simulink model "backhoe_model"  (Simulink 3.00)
settings: Solver=ode4  StartTime=0.0  StopTime=tfinal  FixedStep=T  RelTol=1e-3
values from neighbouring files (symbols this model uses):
  a1 = R(1,1)    [Jacobian.m]    (also in sub_static_vars.m = a(1))
  a2 = R(2,2)    [Jacobian.m]    (also in sub_static_vars.m = a(2))
  a3 = R(3,3)    [Jacobian.m]    (also in sub_static_vars.m = a(3))
  a4 = R(4,1)    [Jacobian.m]    (also in sub_static_vars.m = a(4))
  Ac = pi*(Dc.^2)/4    [cylinders.m]
  Ar = Ac-pi*(Dr.^2)/4    [cylinders.m]
  Cd = 2    [startup.m]
  dt = tfinal/N    (= 0.02)    [demo_trench.m]
  G1 = '0'    [sub_static_vars.m]    (also in symbolic_manip.m = G)
  G2 = char(G{2})    [sub_static_vars.m]    (also in symbolic_manip.m = G)
  G3 = char(G{3})    [sub_static_vars.m]    (also in symbolic_manip.m = G)
  G4 = char(G{4})    [sub_static_vars.m]    (also in symbolic_manip.m = G)
  Lcyl = [12.5*2 25 25.5 21.5]'    [cylinders.m]
  M11 = char(M{1})    [sub_static_vars.m]
  M12 = char(M{2})    [sub_static_vars.m]
  M13 = char(M{3})    [sub_static_vars.m]
  M14 = char(M{4})    [sub_static_vars.m]
  M21 = char(M{5})    [sub_static_vars.m]
  M22 = char(M{6})    [sub_static_vars.m]
  M23 = char(M{7})    [sub_static_vars.m]
  M24 = char(M{8})    [sub_static_vars.m]
  M31 = char(M{9})    [sub_static_vars.m]
  M32 = char(M{10})    [sub_static_vars.m]
  M33 = char(M{11})    [sub_static_vars.m]
  M34 = char(M{12})    [sub_static_vars.m]
  M41 = char(M{13})    [sub_static_vars.m]
  M42 = char(M{14})    [sub_static_vars.m]
  M43 = char(M{15})    [sub_static_vars.m]
  M44 = char(M{16})    [sub_static_vars.m]
  prelief = 2250    [backhoesim.m]
  pT = 0    [backhoesim.m]
  q0 = cyl_to_joint(yc0,R)    [backhoesim.m]
  qmax = cyl_to_joint([yclim(2,1) yclim(2,1) yclim(1,2) yclim(1,3) yclim(1,4)],R)    [backhoesim.m]    (also in demo_trench.m = [1.5708    1.0907    6.1403    6.5025])
  qmin = cyl_to_joint([yclim(1,1) yclim(1,1) yclim(2,2) yclim(2,3) yclim(2,4)],R)    [backhoesim.m]    (also in demo_trench.m = [-1.5708   -0.8529    3.6469    4.1089])
  QP = 33.11    [backhoesim.m]
  R1A = R(1,5)    [cyl_to_joint.m]    (also in dimensions.m = sqrt(R0N^2+(R01-RAN)^2); joint_to_cyl.m; SFr2taur.m; Sjoint_to_cyl.m)
  R1B = R(2,4)    [cyl_to_joint.m]    (also in dimensions.m = 35.875; joint_to_cyl.m; SFr2taur.m; Sjoint_to_cyl.m)
  R2C = R(2,3)    [cyl_to_joint.m]    (also in dimensions.m = 36; joint_to_cyl.m; SFr2taur.m; Sjoint_to_cyl.m)
  R2D = R(3,1)    [cyl_to_joint.m]    (also in dimensions.m = 9.875; joint_to_cyl.m; SFr2taur.m; Sjoint_to_cyl.m)
  R3F = R(3,5)-R(3,7)    [cyl_to_joint.m]    (also in dimensions.m = 4.5; joint_to_cyl.m; SFr2taur.m = R(3,8); Sjoint_to_cyl.m)
  R3G = R(4,2)    [cyl_to_joint.m]    (also in dimensions.m = 5.5; joint_to_cyl.m; SFr2taur.m; Sjoint_to_cyl.m)
  REF = R(3,6)    [cyl_to_joint.m]    (also in dimensions.m = 30.77; joint_to_cyl.m; SFr2taur.m; Sjoint_to_cyl.m)
  RFH = R(4,4)    [cyl_to_joint.m]    (also in dimensions.m = 9.5; joint_to_cyl.m; SFr2taur.m; Sjoint_to_cyl.m)
  RGH = R(4,5)    [cyl_to_joint.m]    (also in dimensions.m = 9.5; joint_to_cyl.m; SFr2taur.m; Sjoint_to_cyl.m)
  T = 0.001    [startup.m]
  T01A = R(1,12)    [cyl_to_joint.m]    (also in dimensions.m = atan(R0N/(R01-RAN)); joint_to_cyl.m; Sjoint_to_cyl.m)
  T12C = R(2,13)    [cyl_to_joint.m]    (also in dimensions.m = acos((R12^2+R2C^2-R1C^2)/(2*R12*R2C)); joint_to_cyl.m; Sjoint_to_cyl.m)
  T23D = acos((R23^2+R3D^2-R2D^2)/(2*R23*R3D))    [cyl_to_joint.m]    (also in dimensions.m; joint_to_cyl.m = R(3,14); SFr2taur.m = R(3,14); Sjoint_to_cyl.m = R(3,14))
  TB12 = R(2,12)    [cyl_to_joint.m]    (also in dimensions.m = acos((R1B^2+R12^2-R2B^2)/(2*R1B*R12)); joint_to_cyl.m; SFr2taur.m; Sjoint_to_cyl.m)
  TD23 = R(3,12)    [cyl_to_joint.m]    (also in dimensions.m = acos((R2D^2+R23^2-R3D^2)/(2*R2D*R23)); joint_to_cyl.m; SFr2taur.m; Sjoint_to_cyl.m)
  TDFE = R(3,13)    [cyl_to_joint.m]    (also in dimensions.m = acos((RDF^2+REF^2-RDE^2)/(2*RDF*REF)); joint_to_cyl.m; SFr2taur.m; Sjoint_to_cyl.m)
  TG34 = R(4,12)    [cyl_to_joint.m]    (also in dimensions.m = acos((R3G^2+R34^2-R4G^2)/(2*R3G*R34)); joint_to_cyl.m; SFr2taur.m; Sjoint_to_cyl.m)
  V1 = char(V{1})    [sub_static_vars.m]    (also in symbolic_manip.m = V)
  V2 = char(V{2})    [sub_static_vars.m]    (also in symbolic_manip.m = V)
  V3 = char(V{3})    [sub_static_vars.m]    (also in symbolic_manip.m = V)
  V4 = char(V{4})    [sub_static_vars.m]    (also in symbolic_manip.m = V)
  yc0 = [21.587 21.587 28.9 45.27 36.195]'    [backhoesim.m]
undefined symbols (not defined in the file or in its folder): Cc, Cr, den, K1, kd, Kr, num, pc0, pr0, td, wn, zeta
libraries: simulink3 x2
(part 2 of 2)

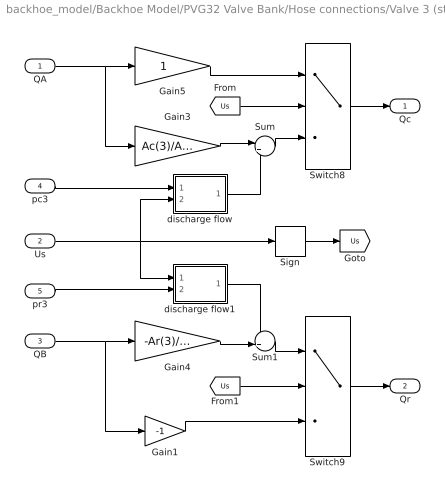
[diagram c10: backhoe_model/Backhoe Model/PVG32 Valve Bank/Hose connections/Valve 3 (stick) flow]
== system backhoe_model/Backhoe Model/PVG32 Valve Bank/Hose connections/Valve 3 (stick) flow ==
  QA : Inport  Port=1  PortWidth=-1  SampleTime=-1  DataType=auto
  Us : Inport  Port=2  PortWidth=-1  SampleTime=-1  DataType=auto
  QB : Inport  Port=3  PortWidth=-1  SampleTime=-1  DataType=auto
  pc3 : Inport  Port=4  PortWidth=-1  SampleTime=-1  DataType=auto
  pr3 : Inport  Port=5  PortWidth=-1  SampleTime=-1  DataType=auto
  Gain1 : Gain  Gain=-1  SaturateOnIntegerOverflow=on
  Gain3 : Gain  Gain=Ac(3)/Ar(3)  SaturateOnIntegerOverflow=on
  Gain4 : Gain  Gain=-Ar(3)/Ac(3)  SaturateOnIntegerOverflow=on
  Gain5 : Gain  Gain=1  SaturateOnIntegerOverflow=on
  Sign : Signum
  Sum : Sum  Inputs=|+-  SaturateOnIntegerOverflow=on
  Sum1 : Sum  Inputs=-+|  SaturateOnIntegerOverflow=on
  Switch8 : Switch  Threshold=0
  Switch9 : Switch  Threshold=0
  discharge flow : Subsystem
  discharge flow1 : Subsystem
  Qc : Outport  Port=1
  Qr : Outport  Port=2
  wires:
  [Us] -> Switch8/2
  Gain5/1 -> Switch8/1
  QA/1 -> Gain3/1, Gain5/1
  Switch8/1 -> Qc/1
  Sum/1 -> Switch8/3
  Gain3/1 -> Sum/1
  [Us] -> Switch9/2
  Gain1/1 -> Switch9/3
  QB/1 -> Gain4/1, Gain1/1
  Switch9/1 -> Qr/1
  Sum1/1 -> Switch9/1
  Gain4/1 -> Sum1/2
  discharge flow/1(Qd) -> Sum/2
  pr3/1 -> discharge flow1/2(p)
  pc3/1 -> discharge flow/1(p)
  Us/1 -> discharge flow/2(Us), discharge flow1/1(Us), Sign/1
  discharge flow1/1(Qd) -> Sum1/1
  Sign/1 -> [Us]

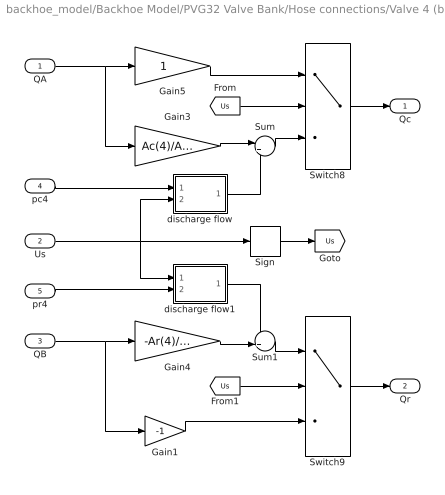
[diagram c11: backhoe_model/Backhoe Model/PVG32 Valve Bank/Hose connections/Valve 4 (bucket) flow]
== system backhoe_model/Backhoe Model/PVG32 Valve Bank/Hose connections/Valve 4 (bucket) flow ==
  QA : Inport  Port=1  PortWidth=-1  SampleTime=-1  DataType=auto
  Us : Inport  Port=2  PortWidth=-1  SampleTime=-1  DataType=auto
  QB : Inport  Port=3  PortWidth=-1  SampleTime=-1  DataType=auto
  pc4 : Inport  Port=4  PortWidth=-1  SampleTime=-1  DataType=auto
  pr4 : Inport  Port=5  PortWidth=-1  SampleTime=-1  DataType=auto
  Gain1 : Gain  Gain=-1  SaturateOnIntegerOverflow=on
  Gain3 : Gain  Gain=Ac(4)/Ar(4)  SaturateOnIntegerOverflow=on
  Gain4 : Gain  Gain=-Ar(4)/Ac(4)  SaturateOnIntegerOverflow=on
  Gain5 : Gain  Gain=1  SaturateOnIntegerOverflow=on
  Sign : Signum
  Sum : Sum  Inputs=|+-  SaturateOnIntegerOverflow=on
  Sum1 : Sum  Inputs=-+|  SaturateOnIntegerOverflow=on
  Switch8 : Switch  Threshold=0
  Switch9 : Switch  Threshold=0
  discharge flow : Subsystem
  discharge flow1 : Subsystem
  Qc : Outport  Port=1
  Qr : Outport  Port=2
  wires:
  [Us] -> Switch8/2
  Gain5/1 -> Switch8/1
  QA/1 -> Gain3/1, Gain5/1
  Switch8/1 -> Qc/1
  Sum/1 -> Switch8/3
  Gain3/1 -> Sum/1
  [Us] -> Switch9/2
  Gain1/1 -> Switch9/3
  QB/1 -> Gain4/1, Gain1/1
  Switch9/1 -> Qr/1
  Sum1/1 -> Switch9/1
  Gain4/1 -> Sum1/2
  pr4/1 -> discharge flow1/2(p)
  Us/1 -> discharge flow/2(Us), discharge flow1/1(Us), Sign/1
  pc4/1 -> discharge flow/1(p)
  discharge flow/1(Qd) -> Sum/2
  discharge flow1/1(Qd) -> Sum1/1
  Sign/1 -> [Us]

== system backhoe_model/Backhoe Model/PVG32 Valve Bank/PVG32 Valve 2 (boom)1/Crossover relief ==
  pR : Inport  Orientation=left  Port=1  PortWidth=-1  SampleTime=-1  DataType=auto
  pL : Inport  Orientation=left  Port=2  PortWidth=-1  SampleTime=-1  DataType=auto
  Q : Inport  Orientation=left  Port=3  PortWidth=-1  SampleTime=-1  DataType=auto
  Gain1 : Gain  Orientation=left  Gain=Kr  SaturateOnIntegerOverflow=on
  MinMax : MinMax  Orientation=left  Function=max  Inputs=2
  Product : Product  Orientation=left  Inputs=3  SaturateOnIntegerOverflow=on
  Relief valve dynamics : TransferFcn  Orientation=left  Numerator=[wn^2]  Denominator=[1 2*zeta*wn wn^2]
  Sum : Sum  Orientation=left  Inputs=|+-  SaturateOnIntegerOverflow=on
  pressure relief threshold : Constant  Orientation=left  Value=prelief
  pump limit : Saturate  Orientation=left  UpperLimit=QP  LowerLimit=0
  valve  cracks open : Relay  Orientation=left  OnSwitchValue=prelief  OffSwitchValue=prelief  OnOutputValue=1  OffOutputValue=0
  Qrelief : Outport  Orientation=left  Port=1
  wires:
  Product/1 -> Gain1/1
  Gain1/1 -> Relief valve dynamics/1
  Relief valve dynamics/1 -> pump limit/1
  Sum/1 -> Product/2
  pressure relief threshold/1 -> Sum/2
  pR/1 -> MinMax/1
  pL/1 -> MinMax/2
  MinMax/1 -> Sum/1, valve  cracks open/1
  pump limit/1 -> Qrelief/1
  Q/1 -> Product/3
  valve  cracks open/1 -> Product/1

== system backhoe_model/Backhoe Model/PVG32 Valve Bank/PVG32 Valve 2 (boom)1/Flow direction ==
  Us : Inport  Port=1  PortWidth=-1  SampleTime=-1  DataType=auto
  Q : Inport  Port=2  PortWidth=-1  SampleTime=-1  DataType=auto
  pA : Inport  Port=3  PortWidth=-1  SampleTime=-1  DataType=auto
  pB : Inport  Port=4  PortWidth=-1  SampleTime=-1  DataType=auto
  Sign : Signum
  Switch{,1..3} (4 alike) : Switch  Threshold=0
  QA : Outport  Port=1
  QB : Outport  Port=2
  pL : Outport  Port=3
  pR : Outport  Port=4
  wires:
  [Us] -> Switch/2
  [Us] -> Switch1/2
  Switch1/1 -> QB/1
  Switch/1 -> QA/1
  Us/1 -> Sign/1
  Sign/1 -> [Us]
  pA/1 -> Switch2/1, Switch3/3
  [Us] -> Switch2/2
  [Us] -> Switch3/2
  pB/1 -> Switch2/3, Switch3/1
  Switch2/1 -> pL/1
  Switch3/1 -> pR/1
  Q/1 -> Switch1/3, Switch/1, Switch1/1, Switch/3

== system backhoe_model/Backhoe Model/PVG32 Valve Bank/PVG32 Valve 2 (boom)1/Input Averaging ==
  Us : Inport  Port=1  PortWidth=-1  SampleTime=-1  DataType=auto
  Abs : Abs
  Integrator : Integrator  ExternalReset=none  InitialConditionSource=internal  InitialCondition=0  LimitOutput=off  UpperSaturationLimit=inf  LowerSaturationLimit=-inf  ShowSaturationPort=off  ShowStatePort=off  AbsoluteTolerance=auto
  Product : Product  Inputs=*/  SaturateOnIntegerOverflow=on
  Sum : Sum  Inputs=|+-  SaturateOnIntegerOverflow=on
  averaging  interval : Constant  Value=dt
  averaging delay : DiscreteTransferFcn  Numerator=[1]  Denominator=[1 zeros(1,kd)]  SampleTime=T
  Ubar : Outport  Port=1
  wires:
  averaging  interval/1 -> Product/2
  Us/1 -> Abs/1
  Abs/1 -> averaging delay/1, Sum/1
  Product/1 -> Ubar/1
  Sum/1 -> Integrator/1
  averaging delay/1 -> Sum/2
  Integrator/1 -> Product/1

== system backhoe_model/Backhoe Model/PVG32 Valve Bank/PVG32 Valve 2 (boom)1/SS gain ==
  note: theoretical Qss
  Ubar : Inport  Port=1  PortWidth=-1  SampleTime=-1  DataType=auto
  " Gain1" : Gain  Gain=34.253  SaturateOnIntegerOverflow=on
  " Gain2" : Gain  Gain=-7.5083  SaturateOnIntegerOverflow=on
  Constant : Constant  Value=1
  Constant1 : Constant  Value=0
  Fcn : Fcn  Expr=u^2
  Gain : Gain  Gain=K1  SaturateOnIntegerOverflow=on
  Product1 : Product  Inputs=*/  SaturateOnIntegerOverflow=on
  Sum1 : Sum  Inputs=+|+|+  SaturateOnIntegerOverflow=on
  Switch : Switch  Threshold=0.001
  Switch1 : Switch  Threshold=0
  intercept : Constant  Value=-0.4345
  Kv : Outport  Port=1
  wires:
  " Gain2"/1 -> Sum1/1
  " Gain1"/1 -> Sum1/2
  intercept/1 -> Sum1/3
  Fcn/1 -> " Gain2"/1
  Constant/1 -> Switch/3
  Switch/1 -> Product1/2
  Product1/1 -> Switch1/1
  Switch1/1 -> Kv/1
  Constant1/1 -> Switch1/3
  Gain/1 -> Product1/1
  Sum1/1 -> Gain/1
  Ubar/1 -> " Gain1"/1, Fcn/1, Switch/2, Switch/1, Switch1/2

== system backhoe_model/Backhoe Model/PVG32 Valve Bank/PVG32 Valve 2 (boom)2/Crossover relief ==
  pR : Inport  Orientation=left  Port=1  PortWidth=-1  SampleTime=-1  DataType=auto
  pL : Inport  Orientation=left  Port=2  PortWidth=-1  SampleTime=-1  DataType=auto
  Q : Inport  Orientation=left  Port=3  PortWidth=-1  SampleTime=-1  DataType=auto
  Gain1 : Gain  Orientation=left  Gain=Kr  SaturateOnIntegerOverflow=on
  MinMax : MinMax  Orientation=left  Function=max  Inputs=2
  Product : Product  Orientation=left  Inputs=3  SaturateOnIntegerOverflow=on
  Relief valve dynamics : TransferFcn  Orientation=left  Numerator=[wn^2]  Denominator=[1 2*zeta*wn wn^2]
  Sum : Sum  Orientation=left  Inputs=|+-  SaturateOnIntegerOverflow=on
  pressure relief threshold : Constant  Orientation=left  Value=prelief
  pump limit : Saturate  Orientation=left  UpperLimit=QP  LowerLimit=0
  valve  cracks open : Relay  Orientation=left  OnSwitchValue=prelief  OffSwitchValue=prelief  OnOutputValue=1  OffOutputValue=0
  Qrelief : Outport  Orientation=left  Port=1
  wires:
  Product/1 -> Gain1/1
  Gain1/1 -> Relief valve dynamics/1
  Relief valve dynamics/1 -> pump limit/1
  Sum/1 -> Product/2
  pressure relief threshold/1 -> Sum/2
  pR/1 -> MinMax/1
  pL/1 -> MinMax/2
  MinMax/1 -> Sum/1, valve  cracks open/1
  pump limit/1 -> Qrelief/1
  Q/1 -> Product/3
  valve  cracks open/1 -> Product/1

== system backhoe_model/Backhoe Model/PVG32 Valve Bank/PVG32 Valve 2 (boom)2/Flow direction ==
  Us : Inport  Port=1  PortWidth=-1  SampleTime=-1  DataType=auto
  Q : Inport  Port=2  PortWidth=-1  SampleTime=-1  DataType=auto
  pA : Inport  Port=3  PortWidth=-1  SampleTime=-1  DataType=auto
  pB : Inport  Port=4  PortWidth=-1  SampleTime=-1  DataType=auto
  Sign : Signum
  Switch{,1..3} (4 alike) : Switch  Threshold=0
  QA : Outport  Port=1
  QB : Outport  Port=2
  pL : Outport  Port=3
  pR : Outport  Port=4
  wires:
  [Us] -> Switch/2
  [Us] -> Switch1/2
  Switch1/1 -> QB/1
  Switch/1 -> QA/1
  Us/1 -> Sign/1
  Sign/1 -> [Us]
  pA/1 -> Switch2/1, Switch3/3
  [Us] -> Switch2/2
  [Us] -> Switch3/2
  pB/1 -> Switch2/3, Switch3/1
  Switch2/1 -> pL/1
  Switch3/1 -> pR/1
  Q/1 -> Switch1/3, Switch/1, Switch1/1, Switch/3

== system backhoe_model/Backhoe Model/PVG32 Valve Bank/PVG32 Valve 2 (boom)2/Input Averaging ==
  Us : Inport  Port=1  PortWidth=-1  SampleTime=-1  DataType=auto
  Abs : Abs
  Integrator : Integrator  ExternalReset=none  InitialConditionSource=internal  InitialCondition=0  LimitOutput=off  UpperSaturationLimit=inf  LowerSaturationLimit=-inf  ShowSaturationPort=off  ShowStatePort=off  AbsoluteTolerance=auto
  Product : Product  Inputs=*/  SaturateOnIntegerOverflow=on
  Sum : Sum  Inputs=|+-  SaturateOnIntegerOverflow=on
  averaging  interval : Constant  Value=dt
  averaging delay : DiscreteTransferFcn  Numerator=[1]  Denominator=[1 zeros(1,kd)]  SampleTime=T
  Ubar : Outport  Port=1
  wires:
  averaging  interval/1 -> Product/2
  Us/1 -> Abs/1
  Abs/1 -> averaging delay/1, Sum/1
  Product/1 -> Ubar/1
  Sum/1 -> Integrator/1
  averaging delay/1 -> Sum/2
  Integrator/1 -> Product/1

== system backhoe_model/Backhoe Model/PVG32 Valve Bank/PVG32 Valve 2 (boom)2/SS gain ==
  note: theoretical Qss
  Ubar : Inport  Port=1  PortWidth=-1  SampleTime=-1  DataType=auto
  " Gain1" : Gain  Gain=34.253  SaturateOnIntegerOverflow=on
  " Gain2" : Gain  Gain=-7.5083  SaturateOnIntegerOverflow=on
  Constant : Constant  Value=1
  Constant1 : Constant  Value=0
  Fcn : Fcn  Expr=u^2
  Gain : Gain  Gain=K1  SaturateOnIntegerOverflow=on
  Product1 : Product  Inputs=*/  SaturateOnIntegerOverflow=on
  Sum1 : Sum  Inputs=+|+|+  SaturateOnIntegerOverflow=on
  Switch : Switch  Threshold=0.001
  Switch1 : Switch  Threshold=0
  intercept : Constant  Value=-0.4345
  Kv : Outport  Port=1
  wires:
  " Gain2"/1 -> Sum1/1
  " Gain1"/1 -> Sum1/2
  intercept/1 -> Sum1/3
  Fcn/1 -> " Gain2"/1
  Constant/1 -> Switch/3
  Switch/1 -> Product1/2
  Product1/1 -> Switch1/1
  Switch1/1 -> Kv/1
  Constant1/1 -> Switch1/3
  Gain/1 -> Product1/1
  Sum1/1 -> Gain/1
  Ubar/1 -> " Gain1"/1, Fcn/1, Switch/2, Switch/1, Switch1/2

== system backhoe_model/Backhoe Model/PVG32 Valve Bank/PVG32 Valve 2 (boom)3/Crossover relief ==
  pR : Inport  Orientation=left  Port=1  PortWidth=-1  SampleTime=-1  DataType=auto
  pL : Inport  Orientation=left  Port=2  PortWidth=-1  SampleTime=-1  DataType=auto
  Q : Inport  Orientation=left  Port=3  PortWidth=-1  SampleTime=-1  DataType=auto
  Gain1 : Gain  Orientation=left  Gain=Kr  SaturateOnIntegerOverflow=on
  MinMax : MinMax  Orientation=left  Function=max  Inputs=2
  Product : Product  Orientation=left  Inputs=3  SaturateOnIntegerOverflow=on
  Relief valve dynamics : TransferFcn  Orientation=left  Numerator=[wn^2]  Denominator=[1 2*zeta*wn wn^2]
  Sum : Sum  Orientation=left  Inputs=|+-  SaturateOnIntegerOverflow=on
  pressure relief threshold : Constant  Orientation=left  Value=prelief
  pump limit : Saturate  Orientation=left  UpperLimit=QP  LowerLimit=0
  valve  cracks open : Relay  Orientation=left  OnSwitchValue=prelief  OffSwitchValue=prelief  OnOutputValue=1  OffOutputValue=0
  Qrelief : Outport  Orientation=left  Port=1
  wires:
  Product/1 -> Gain1/1
  Gain1/1 -> Relief valve dynamics/1
  Relief valve dynamics/1 -> pump limit/1
  Sum/1 -> Product/2
  pressure relief threshold/1 -> Sum/2
  pR/1 -> MinMax/1
  pL/1 -> MinMax/2
  MinMax/1 -> Sum/1, valve  cracks open/1
  pump limit/1 -> Qrelief/1
  Q/1 -> Product/3
  valve  cracks open/1 -> Product/1

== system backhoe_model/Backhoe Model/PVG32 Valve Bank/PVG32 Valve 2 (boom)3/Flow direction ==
  Us : Inport  Port=1  PortWidth=-1  SampleTime=-1  DataType=auto
  Q : Inport  Port=2  PortWidth=-1  SampleTime=-1  DataType=auto
  pA : Inport  Port=3  PortWidth=-1  SampleTime=-1  DataType=auto
  pB : Inport  Port=4  PortWidth=-1  SampleTime=-1  DataType=auto
  Sign : Signum
  Switch{,1..3} (4 alike) : Switch  Threshold=0
  QA : Outport  Port=1
  QB : Outport  Port=2
  pL : Outport  Port=3
  pR : Outport  Port=4
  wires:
  [Us] -> Switch/2
  [Us] -> Switch1/2
  Switch1/1 -> QB/1
  Switch/1 -> QA/1
  Us/1 -> Sign/1
  Sign/1 -> [Us]
  pA/1 -> Switch2/1, Switch3/3
  [Us] -> Switch2/2
  [Us] -> Switch3/2
  pB/1 -> Switch2/3, Switch3/1
  Switch2/1 -> pL/1
  Switch3/1 -> pR/1
  Q/1 -> Switch1/3, Switch/1, Switch1/1, Switch/3

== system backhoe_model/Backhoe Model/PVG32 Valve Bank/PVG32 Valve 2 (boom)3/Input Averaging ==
  Us : Inport  Port=1  PortWidth=-1  SampleTime=-1  DataType=auto
  Abs : Abs
  Integrator : Integrator  ExternalReset=none  InitialConditionSource=internal  InitialCondition=0  LimitOutput=off  UpperSaturationLimit=inf  LowerSaturationLimit=-inf  ShowSaturationPort=off  ShowStatePort=off  AbsoluteTolerance=auto
  Product : Product  Inputs=*/  SaturateOnIntegerOverflow=on
  Sum : Sum  Inputs=|+-  SaturateOnIntegerOverflow=on
  averaging  interval : Constant  Value=dt
  averaging delay : DiscreteTransferFcn  Numerator=[1]  Denominator=[1 zeros(1,kd)]  SampleTime=T
  Ubar : Outport  Port=1
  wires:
  averaging  interval/1 -> Product/2
  Us/1 -> Abs/1
  Abs/1 -> averaging delay/1, Sum/1
  Product/1 -> Ubar/1
  Sum/1 -> Integrator/1
  averaging delay/1 -> Sum/2
  Integrator/1 -> Product/1

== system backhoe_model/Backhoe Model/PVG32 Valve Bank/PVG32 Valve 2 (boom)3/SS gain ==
  note: theoretical Qss
  Ubar : Inport  Port=1  PortWidth=-1  SampleTime=-1  DataType=auto
  " Gain1" : Gain  Gain=34.253  SaturateOnIntegerOverflow=on
  " Gain2" : Gain  Gain=-7.5083  SaturateOnIntegerOverflow=on
  Constant : Constant  Value=1
  Constant1 : Constant  Value=0
  Fcn : Fcn  Expr=u^2
  Gain : Gain  Gain=K1  SaturateOnIntegerOverflow=on
  Product1 : Product  Inputs=*/  SaturateOnIntegerOverflow=on
  Sum1 : Sum  Inputs=+|+|+  SaturateOnIntegerOverflow=on
  Switch : Switch  Threshold=0.001
  Switch1 : Switch  Threshold=0
  intercept : Constant  Value=-0.4345
  Kv : Outport  Port=1
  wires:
  " Gain2"/1 -> Sum1/1
  " Gain1"/1 -> Sum1/2
  intercept/1 -> Sum1/3
  Fcn/1 -> " Gain2"/1
  Constant/1 -> Switch/3
  Switch/1 -> Product1/2
  Product1/1 -> Switch1/1
  Switch1/1 -> Kv/1
  Constant1/1 -> Switch1/3
  Gain/1 -> Product1/1
  Sum1/1 -> Gain/1
  Ubar/1 -> " Gain1"/1, Fcn/1, Switch/2, Switch/1, Switch1/2

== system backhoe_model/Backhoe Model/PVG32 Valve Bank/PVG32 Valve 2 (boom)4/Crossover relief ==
  pR : Inport  Orientation=left  Port=1  PortWidth=-1  SampleTime=-1  DataType=auto
  pL : Inport  Orientation=left  Port=2  PortWidth=-1  SampleTime=-1  DataType=auto
  Q : Inport  Orientation=left  Port=3  PortWidth=-1  SampleTime=-1  DataType=auto
  Gain1 : Gain  Orientation=left  Gain=Kr  SaturateOnIntegerOverflow=on
  MinMax : MinMax  Orientation=left  Function=max  Inputs=2
  Product : Product  Orientation=left  Inputs=3  SaturateOnIntegerOverflow=on
  Relief valve dynamics : TransferFcn  Orientation=left  Numerator=[wn^2]  Denominator=[1 2*zeta*wn wn^2]
  Sum : Sum  Orientation=left  Inputs=|+-  SaturateOnIntegerOverflow=on
  pressure relief threshold : Constant  Orientation=left  Value=prelief
  pump limit : Saturate  Orientation=left  UpperLimit=QP  LowerLimit=0
  valve  cracks open : Relay  Orientation=left  OnSwitchValue=prelief  OffSwitchValue=prelief  OnOutputValue=1  OffOutputValue=0
  Qrelief : Outport  Orientation=left  Port=1
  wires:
  Product/1 -> Gain1/1
  Gain1/1 -> Relief valve dynamics/1
  Relief valve dynamics/1 -> pump limit/1
  Sum/1 -> Product/2
  pressure relief threshold/1 -> Sum/2
  pR/1 -> MinMax/1
  pL/1 -> MinMax/2
  MinMax/1 -> Sum/1, valve  cracks open/1
  pump limit/1 -> Qrelief/1
  Q/1 -> Product/3
  valve  cracks open/1 -> Product/1

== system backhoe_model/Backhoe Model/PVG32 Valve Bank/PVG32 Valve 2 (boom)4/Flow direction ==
  Us : Inport  Port=1  PortWidth=-1  SampleTime=-1  DataType=auto
  Q : Inport  Port=2  PortWidth=-1  SampleTime=-1  DataType=auto
  pA : Inport  Port=3  PortWidth=-1  SampleTime=-1  DataType=auto
  pB : Inport  Port=4  PortWidth=-1  SampleTime=-1  DataType=auto
  Sign : Signum
  Switch{,1..3} (4 alike) : Switch  Threshold=0
  QA : Outport  Port=1
  QB : Outport  Port=2
  pL : Outport  Port=3
  pR : Outport  Port=4
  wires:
  [Us] -> Switch/2
  [Us] -> Switch1/2
  Switch1/1 -> QB/1
  Switch/1 -> QA/1
  Us/1 -> Sign/1
  Sign/1 -> [Us]
  pA/1 -> Switch2/1, Switch3/3
  [Us] -> Switch2/2
  [Us] -> Switch3/2
  pB/1 -> Switch2/3, Switch3/1
  Switch2/1 -> pL/1
  Switch3/1 -> pR/1
  Q/1 -> Switch1/3, Switch/1, Switch1/1, Switch/3

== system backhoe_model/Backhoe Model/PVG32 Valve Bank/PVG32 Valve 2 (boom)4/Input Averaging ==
  Us : Inport  Port=1  PortWidth=-1  SampleTime=-1  DataType=auto
  Abs : Abs
  Integrator : Integrator  ExternalReset=none  InitialConditionSource=internal  InitialCondition=0  LimitOutput=off  UpperSaturationLimit=inf  LowerSaturationLimit=-inf  ShowSaturationPort=off  ShowStatePort=off  AbsoluteTolerance=auto
  Product : Product  Inputs=*/  SaturateOnIntegerOverflow=on
  Sum : Sum  Inputs=|+-  SaturateOnIntegerOverflow=on
  averaging  interval : Constant  Value=dt
  averaging delay : DiscreteTransferFcn  Numerator=[1]  Denominator=[1 zeros(1,kd)]  SampleTime=T
  Ubar : Outport  Port=1
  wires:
  averaging  interval/1 -> Product/2
  Us/1 -> Abs/1
  Abs/1 -> averaging delay/1, Sum/1
  Product/1 -> Ubar/1
  Sum/1 -> Integrator/1
  averaging delay/1 -> Sum/2
  Integrator/1 -> Product/1

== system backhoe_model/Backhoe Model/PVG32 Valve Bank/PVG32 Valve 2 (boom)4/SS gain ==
  note: theoretical Qss
  Ubar : Inport  Port=1  PortWidth=-1  SampleTime=-1  DataType=auto
  " Gain1" : Gain  Gain=34.253  SaturateOnIntegerOverflow=on
  " Gain2" : Gain  Gain=-7.5083  SaturateOnIntegerOverflow=on
  Constant : Constant  Value=1
  Constant1 : Constant  Value=0
  Fcn : Fcn  Expr=u^2
  Gain : Gain  Gain=K1  SaturateOnIntegerOverflow=on
  Product1 : Product  Inputs=*/  SaturateOnIntegerOverflow=on
  Sum1 : Sum  Inputs=+|+|+  SaturateOnIntegerOverflow=on
  Switch : Switch  Threshold=0.001
  Switch1 : Switch  Threshold=0
  intercept : Constant  Value=-0.4345
  Kv : Outport  Port=1
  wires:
  " Gain2"/1 -> Sum1/1
  " Gain1"/1 -> Sum1/2
  intercept/1 -> Sum1/3
  Fcn/1 -> " Gain2"/1
  Constant/1 -> Switch/3
  Switch/1 -> Product1/2
  Product1/1 -> Switch1/1
  Switch1/1 -> Kv/1
  Constant1/1 -> Switch1/3
  Gain/1 -> Product1/1
  Sum1/1 -> Gain/1
  Ubar/1 -> " Gain1"/1, Fcn/1, Switch/2, Switch/1, Switch1/2

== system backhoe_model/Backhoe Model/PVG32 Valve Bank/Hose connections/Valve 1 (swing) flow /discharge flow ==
  p : Inport  Port=1  PortWidth=-1  SampleTime=-1  DataType=auto
  Us : Inport  Port=2  PortWidth=-1  SampleTime=-1  DataType=auto
  Abs : Abs
  Fcn : Fcn  Expr=sqrt(u)
  Product : Product  Inputs=2  SaturateOnIntegerOverflow=on
  discharge coeff : Gain  Gain=Cd  SaturateOnIntegerOverflow=on
  Qd : Outport  Port=1
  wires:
  Us/1 -> Abs/1
  p/1 -> Fcn/1
  Abs/1 -> Product/1
  Fcn/1 -> Product/2
  Product/1 -> discharge coeff/1
  discharge coeff/1 -> Qd/1

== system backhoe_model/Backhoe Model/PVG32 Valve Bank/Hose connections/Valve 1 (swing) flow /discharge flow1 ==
  Us : Inport  Port=1  PortWidth=-1  SampleTime=-1  DataType=auto
  p : Inport  Port=2  PortWidth=-1  SampleTime=-1  DataType=auto
  Abs : Abs
  Fcn : Fcn  Expr=sqrt(u)
  Product : Product  Inputs=2  SaturateOnIntegerOverflow=on
  discharge coeff : Gain  Gain=Cd  SaturateOnIntegerOverflow=on
  Qd : Outport  Port=1
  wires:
  Us/1 -> Abs/1
  p/1 -> Fcn/1
  Abs/1 -> Product/1
  Fcn/1 -> Product/2
  Product/1 -> discharge coeff/1
  discharge coeff/1 -> Qd/1

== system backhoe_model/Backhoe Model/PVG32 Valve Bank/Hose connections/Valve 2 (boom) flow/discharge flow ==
  p : Inport  Port=1  PortWidth=-1  SampleTime=-1  DataType=auto
  Us : Inport  Port=2  PortWidth=-1  SampleTime=-1  DataType=auto
  Abs : Abs
  Fcn : Fcn  Expr=sqrt(u)
  Product : Product  Inputs=2  SaturateOnIntegerOverflow=on
  discharge coeff : Gain  Gain=Cd  SaturateOnIntegerOverflow=on
  Qd : Outport  Port=1
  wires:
  Us/1 -> Abs/1
  p/1 -> Fcn/1
  Abs/1 -> Product/1
  Fcn/1 -> Product/2
  Product/1 -> discharge coeff/1
  discharge coeff/1 -> Qd/1

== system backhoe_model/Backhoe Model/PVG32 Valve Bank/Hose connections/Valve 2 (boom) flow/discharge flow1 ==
  Us : Inport  Port=1  PortWidth=-1  SampleTime=-1  DataType=auto
  p : Inport  Port=2  PortWidth=-1  SampleTime=-1  DataType=auto
  Abs : Abs
  Fcn : Fcn  Expr=sqrt(u)
  Product : Product  Inputs=2  SaturateOnIntegerOverflow=on
  discharge coeff : Gain  Gain=Cd  SaturateOnIntegerOverflow=on
  Qd : Outport  Port=1
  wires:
  Us/1 -> Abs/1
  p/1 -> Fcn/1
  Abs/1 -> Product/1
  Fcn/1 -> Product/2
  Product/1 -> discharge coeff/1
  discharge coeff/1 -> Qd/1

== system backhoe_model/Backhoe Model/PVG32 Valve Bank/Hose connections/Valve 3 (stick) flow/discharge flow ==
  p : Inport  Port=1  PortWidth=-1  SampleTime=-1  DataType=auto
  Us : Inport  Port=2  PortWidth=-1  SampleTime=-1  DataType=auto
  Abs : Abs
  Fcn : Fcn  Expr=sqrt(u)
  Product : Product  Inputs=2  SaturateOnIntegerOverflow=on
  discharge coeff : Gain  Gain=Cd  SaturateOnIntegerOverflow=on
  Qd : Outport  Port=1
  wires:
  Us/1 -> Abs/1
  p/1 -> Fcn/1
  Abs/1 -> Product/1
  Fcn/1 -> Product/2
  Product/1 -> discharge coeff/1
  discharge coeff/1 -> Qd/1

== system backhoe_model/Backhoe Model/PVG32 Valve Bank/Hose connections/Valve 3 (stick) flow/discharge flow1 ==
  Us : Inport  Port=1  PortWidth=-1  SampleTime=-1  DataType=auto
  p : Inport  Port=2  PortWidth=-1  SampleTime=-1  DataType=auto
  Abs : Abs
  Fcn : Fcn  Expr=sqrt(u)
  Product : Product  Inputs=2  SaturateOnIntegerOverflow=on
  discharge coeff : Gain  Gain=Cd  SaturateOnIntegerOverflow=on
  Qd : Outport  Port=1
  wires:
  Us/1 -> Abs/1
  p/1 -> Fcn/1
  Abs/1 -> Product/1
  Fcn/1 -> Product/2
  Product/1 -> discharge coeff/1
  discharge coeff/1 -> Qd/1

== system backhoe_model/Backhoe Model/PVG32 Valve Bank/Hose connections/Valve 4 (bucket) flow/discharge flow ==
  p : Inport  Port=1  PortWidth=-1  SampleTime=-1  DataType=auto
  Us : Inport  Port=2  PortWidth=-1  SampleTime=-1  DataType=auto
  Abs : Abs
  Fcn : Fcn  Expr=sqrt(u)
  Product : Product  Inputs=2  SaturateOnIntegerOverflow=on
  discharge coeff : Gain  Gain=Cd  SaturateOnIntegerOverflow=on
  Qd : Outport  Port=1
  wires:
  Us/1 -> Abs/1
  p/1 -> Fcn/1
  Abs/1 -> Product/1
  Fcn/1 -> Product/2
  Product/1 -> discharge coeff/1
  discharge coeff/1 -> Qd/1

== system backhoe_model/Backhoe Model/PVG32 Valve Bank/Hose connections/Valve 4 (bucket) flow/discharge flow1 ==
  Us : Inport  Port=1  PortWidth=-1  SampleTime=-1  DataType=auto
  p : Inport  Port=2  PortWidth=-1  SampleTime=-1  DataType=auto
  Abs : Abs
  Fcn : Fcn  Expr=sqrt(u)
  Product : Product  Inputs=2  SaturateOnIntegerOverflow=on
  discharge coeff : Gain  Gain=Cd  SaturateOnIntegerOverflow=on
  Qd : Outport  Port=1
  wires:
  Us/1 -> Abs/1
  p/1 -> Fcn/1
  Abs/1 -> Product/1
  Fcn/1 -> Product/2
  Product/1 -> discharge coeff/1
  discharge coeff/1 -> Qd/1
